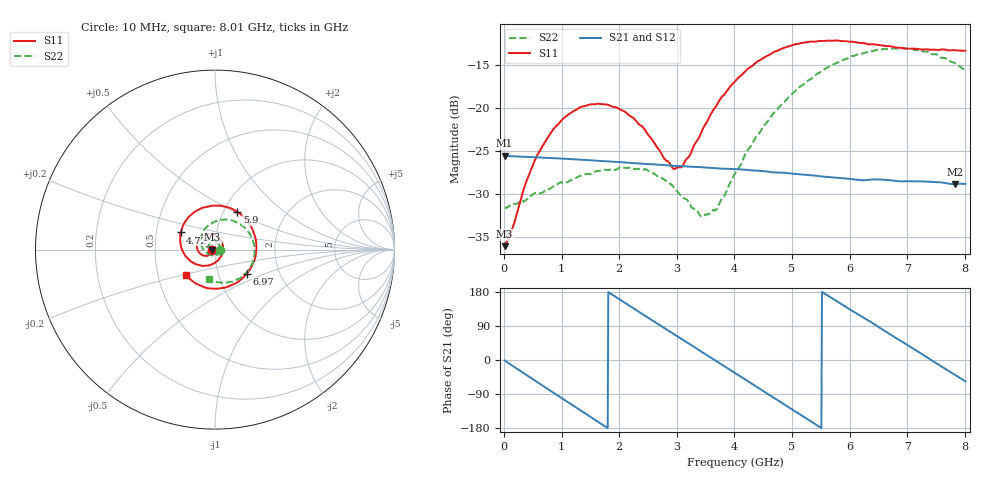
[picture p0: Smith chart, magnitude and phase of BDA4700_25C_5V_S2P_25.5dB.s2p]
!Agilent Technologies,E5071B,MY42404982,A.09.10
!Date: Mon Oct 20 13:39:19 2025
!Data & Calibration Information:
!Freq	S11:SOLT2(ON)	S21:SOLT2(ON)	S12:SOLT2(ON)	S22:SOLT2(ON)
# Hz S RI R 50
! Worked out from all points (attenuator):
!   801 points, 10 MHz to 8.01 GHz, reference 50 ohm
!   highest |S21| = -25.58 dB at 10 MHz (marker M1); lowest = -28.9 dB at 7.83 GHz (marker M2)
!   lowest |S11| = -36.1 dB at 10 MHz (marker M3), VSWR 1.03, Z = 48.5 - j0.122 ohm
!   |S11| at or under -10 dB: start of sweep to end of sweep
!   |S22| runs from -32.7 to -13.0 dB; largest |S21 - S12| = 0.00046
!   S11 on the Smith chart (normalised r, x): 10 MHz: 0.97, -0.00; 4.72 GHz: 0.67, +0.13; 5.9 GHz: 1.16, +0.52; 6.97 GHz: 1.37, -0.38; 8.01 GHz: 0.70, -0.21
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1e7  -0.0156 -0.00125  0.0526 -0.00112  0.0526 -0.00117  0.0261 -0.000842
1.3e8  -0.0167 -0.00932  0.0508 -0.0121  0.0508 -0.0122  0.0266 -0.00625
3.7e8  -0.0257 -0.0249  0.041 -0.0316  0.0411 -0.0317  0.0216 -0.019
6e8  -0.0425 -0.0344  0.0252 -0.0448  0.0251 -0.0448  0.0128 -0.0291
1e9  -0.0812 -0.0239  -0.00925 -0.0497  -0.00923 -0.0498  -0.0146 -0.0338
1.35e9  -0.101 0.0113  -0.0354 -0.035  -0.0354 -0.0351  -0.036 -0.0178
2.07e9  -0.0457 0.0844  -0.0431 0.0213  -0.0432 0.0213  -0.0304 0.0332
2.68e9  0.0346 0.0461  -0.00346 0.0465  -0.00344 0.0465  0.0129 0.0374
2.93e9  0.044 0.00583  0.0158 0.0432  0.0157 0.0432  0.0248 0.0246
3.06e9  0.0417 -0.017  0.0246 0.0386  0.0244 0.0386  0.0274 0.0147
3.44e9  -0.00187 -0.0739  0.0422 0.016  0.0422 0.016  0.0185 -0.014
3.69e9  -0.0514 -0.0898  0.0444 -0.00252  0.0444 -0.00272  0.000467 -0.0256
4.01e9  -0.1226 -0.0725  0.0363 -0.0248  0.0363 -0.0247  -0.0322 -0.0257
4.72e9  -0.1913 0.0957  -0.00961 -0.0408  -0.00952 -0.041  -0.0796 0.0541
5.35e9  -0.0593 0.2357  -0.0389 -0.0111  -0.0388 -0.0112  -0.0155 0.1479
5.9e9  0.1251 0.2099  -0.0313 0.0231  -0.0312 0.0231  0.1073 0.1576
6.27e9  0.2094 0.1112  -0.0127 0.0357  -0.0124 0.0358  0.1832 0.1016
6.68e9  0.2254 -0.0383  0.013 0.0357  0.0131 0.0356  0.2199 -9.27e-05
6.97e9  0.1768 -0.1332  0.0274 0.0255  0.0274 0.0253  0.2075 -0.0777
7.4e9  0.041 -0.2139  0.0371 0.00113  0.0372 0.000997  0.1285 -0.1633
7.83e9  -0.1134 -0.1847  0.028 -0.0225  0.028 -0.0226  0.013 -0.1815
8.01e9  -0.1628 -0.1411  0.0201 -0.0299  0.0202 -0.0299  -0.0307 -0.162
